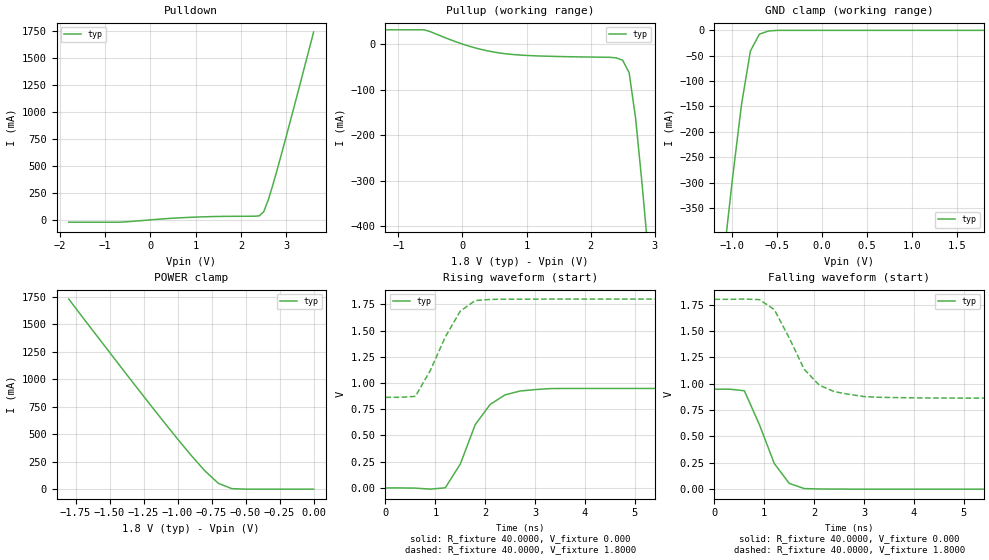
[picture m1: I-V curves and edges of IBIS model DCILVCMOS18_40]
| / 7\'7
| \ \   Xilinx Inc.
| / /
| \_\/.\   IBIS Model for Virtex-II
[IBIS ver]   2.1
[File name]   dci1840.ibs
[File Rev]   1.1
[Date]   Aug. 1, 2001
[Source]   Hspice simulations (08-01: TT, SS, FF)
[Notes]   Xilinx IBIS model for LVDCI 1.8V 40 ohms driver
[Disclaimer] The data in this model is derived from SPICE simulations using
   modeling information extracted from the target process. While
   a great deal of care has been taken to provide information
   that is accurate, this model is considered preliminary as it
   has not been verified by actual silicon measurement. Treat the
   data in this model as preliminary until actual silicon
   verification is performed.
[Copyright]   Copyright 2001, Xilinx Inc., All rights reserved
|   Component Virtex_II
[Component]   Virtex_II
[Manufacturer]   Xilinx Inc.
[Package]
| variable   typ   min   max
R_pkg   0.1000   NA   NA
L_pkg   0.8000nH   NA   NA
C_pkg   0.5000pF   NA   NA
[Pin]  signal_name   model_name   R_pin   L_pin   C_pin
io   DCILVCMOS18_40   DCILVCMOS18_40
| ins  insig   inp
| ens  ensig   inp
PGND   GND   GND
VCCO   VCCO   POWER
| Models and submodels in the file (1): DCILVCMOS18_40 (I/O)
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|   Model DCILVCMOS18_40
[Model]   DCILVCMOS18_40
Model_type   I/O
Polarity   Non-Inverting
Enable   Active-Low
Vinh = 1.19V
Vinl = 0.4V
Vmeas =   0.7900V
Cref =  35.0000pF
Rref =   1.0000M
Vref =  0.000V
C_comp   7.0000pF   NA   NA
[Temperature Range]   25.0000   NA   NA
[Voltage Range]   1.8000V   NA   NA
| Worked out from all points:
|   slope of the pulldown table from 0 to 0.27 V, typ, clamps not added: 30.2 ohm
|   slope of the pullup table from 0 to 0.27 V, typ, clamps not added: 24.6 ohm
|   GND clamp passes 1 mA (typ) near -0.57 V on its own axis
|   POWER clamp passes 1 mA (typ) near -0.52 V on its own axis
|   rising waveform, R_fixture 40.0000, V_fixture 0.000: 20-80 % time 591ps typ, NA min, NA max; typ from 0 V to 0.948 V
|   rising waveform, R_fixture 40.0000, V_fixture 1.8000: 20-80 % time 595ps typ, NA min, NA max; typ from 0.864 V to 1.8 V
|   falling waveform, R_fixture 40.0000, V_fixture 0.000: 20-80 % time 522ps typ, NA min, NA max; typ from 0.948 V to 0 V
|   falling waveform, R_fixture 40.0000, V_fixture 1.8000: 20-80 % time 671ps typ, NA min, NA max; typ from 1.8 V to 0.864 V
[Pulldown]
| voltage   I(typ)   I(min)   I(max)
-1.8V     -21.54mA   NA         NA
-700mV    -21.54mA   NA         NA
900mV     24.08mA    NA         NA
2.4V      36.97mA    NA         NA
2.5V      75.31mA    NA         NA
2.6V      184.1mA    NA         NA
2.7V      322.1mA    NA         NA
3V        780.2mA    NA         NA
3.6V      1.743A     NA         NA
[Pullup]
| voltage   I(typ)   I(min)   I(max)
-1.8V     31.33mA    NA         NA
-600mV    31.33mA    NA         NA
100mV     -4.464mA   NA         NA
600mV     -20.01mA   NA         NA
1.1V      -25.66mA   NA         NA
2.3V      -29.13mA   NA         NA
2.5V      -35.71mA   NA         NA
2.6V      -62.88mA   NA         NA
2.7V      -162.2mA   NA         NA
2.8V      -304.9mA   NA         NA
2.9V      -462.6mA   NA         NA
3.6V      -1.658A    NA         NA
[GND_clamp]
| voltage   I(typ)   I(min)   I(max)
-1.8V     -1.649A    NA         NA
-1.1V     -452.1mA   NA         NA
-1V       -293.4mA   NA         NA
-900mV    -148mA     NA         NA
-800mV    -41.01mA   NA         NA
-700mV    -7.602mA   NA         NA
-600mV    -1.419mA   NA         NA
-500mV    -128.9uA   NA         NA
1.8V      272.1nA    NA         NA
[POWER_clamp]
| voltage   I(typ)   I(min)   I(max)
-1.8V     1.731A     NA         NA
-1.4V     1.085A     NA         NA
-1V       456.9mA    NA         NA
-800mV    167.8mA    NA         NA
-700mV    52.78mA    NA         NA
-600mV    4.607mA    NA         NA
0V        272.1nA    NA         NA
[Ramp]
| variable   typ   min   max
dV/dt_r   0.5690/0.6206n   NA   NA
dV/dt_f   0.5618/0.7239n   NA   NA
R_load = 40.0000
[Rising Waveform]
R_fixture = 40.0000
V_fixture = 0.000
| time   V(typ)   V(min)   V(max)
0s        6.403uV    NA         NA
900ps     -11.78mV   NA         NA
1.2ns     1.417mV    NA         NA
1.5ns     227.4mV    NA         NA
1.8ns     604mV      NA         NA
2.1ns     796.6mV    NA         NA
2.4ns     887.3mV    NA         NA
2.7ns     923.8mV    NA         NA
3.6ns     948.2mV    NA         NA
15ns      948.3mV    NA         NA
[Rising Waveform]
R_fixture = 40.0000
V_fixture = 1.8000
V_fixture_min = 1.7000
V_fixture_max = 1.9000
| time   V(typ)   V(min)   V(max)
0s        863.6mV    NA         NA
300ps     863.6mV    NA         NA
600ps     873mV      NA         NA
900ps     1.12V      NA         NA
1.2ns     1.44V      NA         NA
1.5ns     1.685V     NA         NA
1.8ns     1.786V     NA         NA
2.1ns     1.796V     NA         NA
3.3ns     1.8V       NA         NA
15ns      1.8V       NA         NA
[Falling Waveform]
R_fixture = 40.0000
V_fixture = 0.000
| time   V(typ)   V(min)   V(max)
0s        948.4mV    NA         NA
300ps     948.3mV    NA         NA
600ps     933.1mV    NA         NA
900ps     613.5mV    NA         NA
1.2ns     243.4mV    NA         NA
1.5ns     54.75mV    NA         NA
1.8ns     5.899mV    NA         NA
3ns       222.7uV    NA         NA
15ns      -13.91uV   NA         NA
[Falling Waveform]
R_fixture = 40.0000
V_fixture = 1.8000
V_fixture_min = 1.7000
V_fixture_max = 1.9000
| time   V(typ)   V(min)   V(max)
0s        1.8V       NA         NA
900ps     1.798V     NA         NA
1.2ns     1.703V     NA         NA
1.5ns     1.433V     NA         NA
1.8ns     1.137V     NA         NA
2.1ns     986.6mV    NA         NA
2.4ns     925.1mV    NA         NA
3ns       878.1mV    NA         NA
4.8ns     863.9mV    NA         NA
15ns      863.6mV    NA         NA
